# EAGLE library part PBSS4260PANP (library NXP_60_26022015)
60 V, 2 A NPN/PNP low VCEsat (BISS) transistor NPN/PNP low VCEsat Breakthrough In Small Signal (BISS) transistor in a leadless medium power DFN2020-6 (SOT1118) Surface-Mounted Device (SMD) plastic package. NPN/NPN complement: PBSS4260PAN. PNP/PNP complement: PBSS5260PAP. AAL Eindhoven MK
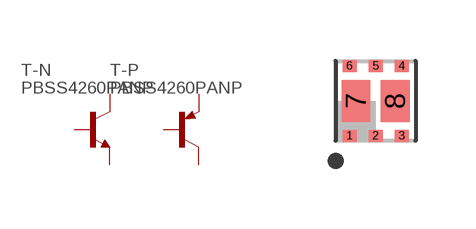
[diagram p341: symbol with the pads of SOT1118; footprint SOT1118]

Designator prefix T; gates -P=PNP -N=NPN

## PBSS4260PANP  [SOT1118]
1  -N:E  pas
2  -N:B  pas
3  -P:C  pas
4  -P:E  pas
5  -P:B  pas
6  -N:C  pas
7  -N:C  pas
8  -P:C  pas

## Footprint SOT1118 (pad centres in mm)
SOT1118 HUSON6: plastic, thermal enhanced ultra thin small outline package; no leads;6 terminals; body 2 x 2 x 0.65 mm JEDEC: -- IEC: -- JEITA: --
smd 0.35 x 0.3: 1 -0.65,-0.875; 2 0,-0.875; 3 0.65,-0.875; 4 0.65,0.875; 5 0,0.875; 6 -0.65,0.875
smd 0.72 x 1.05: 7 -0.49,0; 8 0.49,0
